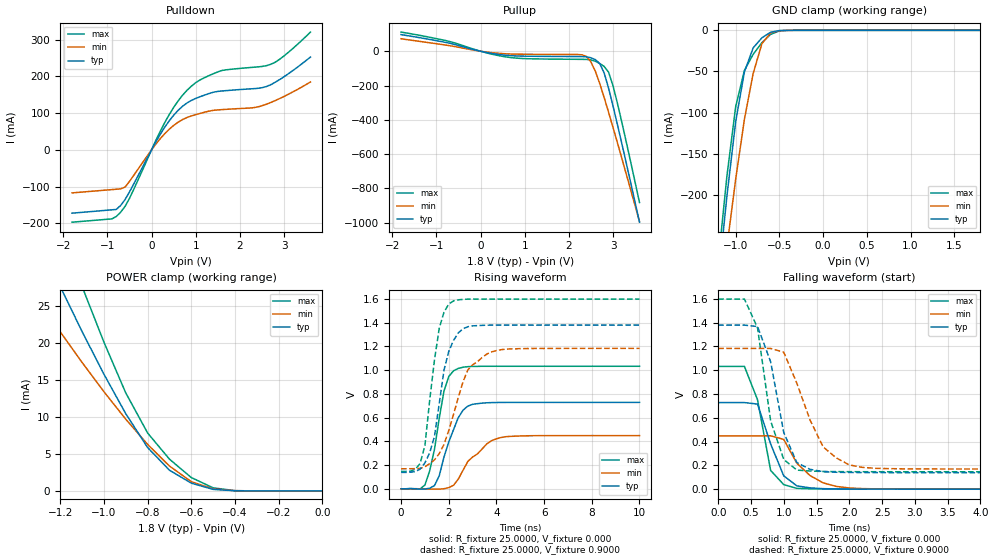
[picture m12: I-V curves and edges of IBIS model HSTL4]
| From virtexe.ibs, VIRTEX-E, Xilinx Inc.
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|   Model HSTL4
[Model]   HSTL4
Model_type   I/O
Polarity   Non-Inverting
Enable   Active-Low
Vmeas =   0.9000V
Vinl =  0.8000V
Vinh =  1.0000V
Cref =  20.0000pF
Rref =  25.0000
Vref =   0.9000V
C_comp   6.0000pF   5.0000pF   7.0000pF
[Temperature Range]   25.0000   100.0000   0.000
[Voltage Range]   1.8000V   1.7000V   1.9000V
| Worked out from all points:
|   slope of the pulldown table from 0 to 0.27 V, typ, clamps not added: 4.8 ohm
|   slope of the pullup table from 0 to 0.27 V, typ, clamps not added: 20.1 ohm
|   GND clamp passes 1 mA (typ) near -0.54 V on its own axis
|   POWER clamp passes 1 mA (typ) near -0.59 V on its own axis
|   rising waveform, R_fixture 25.0000, V_fixture 0.000: 20-80 % time 721ps typ, 1.08ns min, 542ps max; typ from 0 V to 0.728 V
|   rising waveform, R_fixture 25.0000, V_fixture 0.9000: 20-80 % time 646ps typ, 964ps min, 530ps max; typ from 0.138 V to 1.38 V
|   falling waveform, R_fixture 25.0000, V_fixture 0.000: 20-80 % time 295ps typ, 422ps min, 236ps max; typ from 0.728 V to 0 V
|   falling waveform, R_fixture 25.0000, V_fixture 0.9000: 20-80 % time 311ps typ, 455ps min, 272ps max; typ from 1.38 V to 0.138 V
[Pulldown]
| voltage   I(typ)   I(min)   I(max)
-1.8V     -172.5mA   -117.3mA   -197.1mA
-900mV    -163.4mA   -108.3mA   -188.2mA
-700mV    -151.6mA   -106.3mA   -169.9mA
-500mV    -114.8mA   -86.09mA   -132.3mA
300mV     61.93mA    44.24mA    74.52mA
700mV     118.5mA    82.37mA    148.5mA
1V        140.1mA    95.93mA    183mA
1.6V      160.5mA    109.7mA    216.5mA
2.3V      166.6mA    114.8mA    225mA
2.7V      177.5mA    129mA      233.1mA
3V        199.2mA    145.5mA    255.9mA
3.6V      253mA      185mA      320.9mA
[Pullup]
| voltage   I(typ)   I(min)   I(max)
-1.8V     97.04mA    72.78mA    111.7mA
-800mV    51.88mA    36.3mA     62.98mA
600mV     -24.24mA   -15.32mA   -34.04mA
2.3V      -31.3mA    -20.95mA   -47.36mA
2.4V      -32.73mA   -30.87mA   -47.8mA
2.6V      -49.01mA   -116.6mA   -58.63mA
2.7V      -71.91mA   -188.9mA   -71.8mA
2.8V      -127.2mA   -270.6mA   -88.68mA
2.9V      -216mA     -356.6mA   -122.6mA
3V        -319mA     -444.8mA   -201.1mA
3.2V      -539.1mA   -625.1mA   -414.5mA
3.6V      -997.5mA   -993.6mA   -882.6mA
[GND_clamp]
| voltage   I(typ)   I(min)   I(max)
-1.8V     -984.2mA   -893.8mA   -981.3mA
-1.2V     -305.4mA   -349.4mA   -281.7mA
-1.1V     -201.6mA   -263.3mA   -177.2mA
-1V       -111.1mA   -181.2mA   -92.91mA
-900mV    -50.62mA   -108.2mA   -48.68mA
-800mV    -21.39mA   -52.51mA   -29.19mA
-700mV    -9.057mA   -16.26mA   -15mA
-600mV    -2.332mA   -3.044mA   -4.887mA
-500mV    -280.5uA   -493uA     -684.1uA
-400mV    -21.31uA   -72.94uA   -46.93uA
1.8V      9.75nA     24.68nA    9.371nA
[POWER_clamp]
| voltage   I(typ)   I(min)   I(max)
-1.8V     67.36mA    47.92mA    87.19mA
-1.3V     33.96mA    25.81mA    43.76mA
-1.2V     27.64mA    21.52mA    35.56mA
-1.1V     21.56mA    17.38mA    27.65mA
-1V       15.79mA    13.42mA    20.13mA
-900mV    10.45mA    9.702mA    13.26mA
-800mV    5.872mA    6.297mA    7.84mA
-700mV    2.804mA    3.371mA    4.298mA
-600mV    1.052mA    1.252mA    1.806mA
-500mV    210uA      278.7uA    420.1uA
-400mV    17.08uA    35.57uA    36.55uA
0V        9.75nA     16.07nA    10.24nA
[Ramp]
| variable   typ   min   max
dV/dt_r   0.4367/0.7104n   0.2689/1.0764n   0.6192/0.5033n
dV/dt_f   0.9052/0.3522n   0.7960/0.5601n   0.9836/0.2799n
R_load = 25.0000
[Rising Waveform]
R_fixture = 25.0000
V_fixture = 0.000
| time   V(typ)   V(min)   V(max)
0s        0V         0V         632.3nV
1ns       -1.851mV   -1.513mV   32.48mV
1.4ns     26.86mV    -3.036mV   331.7mV
1.6ns     110.2mV    -2.414mV   594.4mV
1.8ns     268.2mV    712.3uV    824.3mV
2ns       395.1mV    10.19mV    946.2mV
2.2ns     498.3mV    29.5mV     993.8mV
2.8ns     696.8mV    230.6mV    1.029V
4.2ns     727.4mV    432.4mV    1.032V
10ns      727.9mV    448.1mV    1.032V
[Rising Waveform]
R_fixture = 25.0000
V_fixture = 0.9000
V_fixture_min = 0.8300
V_fixture_max = 1.1000
| time   V(typ)   V(min)   V(max)
0s        138.4mV    168.8mV    146.2mV
800ps     166mV      171.4mV    214mV
1ns       218.6mV    185.6mV    366.3mV
1.4ns     441.2mV    243.8mV    1.085V
1.6ns     717.8mV    296.5mV    1.352V
1.8ns     1V         374.5mV    1.488V
2ns       1.157V     492.1mV    1.556V
2.8ns     1.365V     1.001V     1.597V
3.8ns     1.379V     1.153V     1.598V
10ns      1.379V     1.183V     1.598V
[Falling Waveform]
R_fixture = 25.0000
V_fixture = 0.000
| time   V(typ)   V(min)   V(max)
0s        727.9mV    448.2mV    1.032V
400ps     727.9mV    448.2mV    1.032V
600ps     715.1mV    448mV      751.3mV
800ps     379.7mV    448.8mV    157.4mV
1ns       111.6mV    418.1mV    38.01mV
1.2ns     27.68mV    217.8mV    6.72mV
1.4ns     10.94mV    114.8mV    3.329mV
1.6ns     4.133mV    53.29mV    1.524mV
2.2ns     802.9uV    4.792mV    443.1uV
10ns      40.54uV    60.3uV     44.11uV
[Falling Waveform]
R_fixture = 25.0000
V_fixture = 0.9000
V_fixture_min = 0.8300
V_fixture_max = 1.1000
| time   V(typ)   V(min)   V(max)
0s        1.379V     1.183V     1.598V
400ps     1.379V     1.183V     1.598V
600ps     1.367V     1.183V     1.357V
800ps     1.071V     1.183V     573.8mV
1ns       475.6mV    1.151V     249.5mV
1.2ns     223.6mV    890.4mV    160.3mV
1.4ns     166.8mV    582.7mV    152.5mV
1.6ns     147.3mV    355.7mV    148.7mV
2.2ns     139.6mV    183.1mV    146.7mV
10ns      138.4mV    168.9mV    146.2mV
